| IBIS file generated by GenIBIS.pl Version 3.07
|   am35xxzcn
[IBIS ver]   4.1
[File name]   sprm451.ibs
[File Rev]   1.0
[Date]   Mon May 10, 2010, 10:46:0
[Source]   Data created at Texas Instruments
[Notes]   1) IBIS spec conformance checker (IBISCK4) ran with 0 errors
   and 179 warnings.  Warnings can be waived.
[Disclaimer] Please be aware that in the absence of a written agreement,
   Texas Instruments (TI) assumes no liability for: 1) the
   accuracy of the IBIS models provided to your company, 2) the
   proper functioning of these IBIS models in your design or for
   any resulting applications, or, 3) infringement of patents,
   copyrights, or intellectual property rights resulting from
   your use of these IBIS models. TI provides IBIS models as a
   service to our customers and therefore reserves the right to
   limit distribution of the IBIS models.
[Copyright]   Property of Texas Instruments Incorporated. Unauthorised
   reproduction and/or distribution is strictly prohibited. This
   product is protected under copyright law and trade secret law
   as an unpublished work. Created 2010,(C) Copyright 2010,
   Texas Instruments Incorporated., All Rights Reserved. These
   commodities are under the U.S. Government distribution license
   control.As such,they are not to be re-exported without the
   prior approval of the U.S. Department of Commerce.
|   Component am35xxzcn
[Component]   am35xxzcn
[Manufacturer]   Texas Instruments.
[Package Model] am35xxzcn
[Package]
|   typ   min   max
R_pkg   0.6975   3.15E-1   1.08E0
L_pkg   3.5033E-009   2.66E-11   6.98E-9
C_pkg   6.86115E-013   2.23E-15   1.37E-12
[Pin]   signal_name   model_name
A2   SDRC_DQS3P   Selector_16
A3   SDRC_D25   Selector_16
A4   SDRC_STRBEN_DLY1   Selector_16
A5   SDRC_STRBEN1   Selector_3
A6   SDRC_DQS2P   Selector_16
A7   SDRC_D16   Selector_16
A8   SDRC_A12   Selector_27
A9   SDRC_A10   Selector_27
A10   SDRC_A5   Selector_27
A11   SDRC_A0   Selector_27
A12   SDRC_BA0   Selector_27
A13   SDRC_CLK   Selector_27
A14   SDRC_NCS1   Selector_27
A15   SDRC_D15   Selector_16
A16   SDRC_D14   Selector_16
A17   SDRC_DQS1N   Selector_16
A18   SDRC_STRBEN_DLY0   Selector_16
A19   SDRC_STRBEN0   Selector_3
A20   SDRC_DQS0N   Selector_16
A21   SDRC_D1   Selector_16
A22   MCBSP4_FSX   Selector_25
A23   MCBSP4_DR   Selector_25
A24   MCBSP3_CLKX   Selector_25
AA1   SYS_BOOT1   Selector_26
AA2   SYS_BOOT2   Selector_26
AA3   SYS_BOOT3   Selector_26
AA7   RMII_RXD1   Selector_12
AA9   MMC1_CLK   Selector_25
AA10   MMC1_DAT3   Selector_25
AA16   MCSPI2_CS0   Selector_4
AA18   ETK_D3   Selector_8
AA19   UART1_TX   Selector_25
AA23   DSS_DATA7   Selector_8
AA24   DSS_DATA8   Selector_8
AA25   DSS_DATA9   Selector_8
AB1   SYS_BOOT4   Selector_26
AB2   SYS_BOOT5   Selector_26
AB6   CCDC_DATA6   Selector_25
AB7   RMII_CRS_DV   Selector_12
AB9   MMC1_CMD   Selector_25
AB10   MMC1_DAT4   Selector_25
AB12   MMC2_DAT0   Selector_12
AB13   MMC2_DAT4   Selector_25
AB15   MCSPI1_CS0   Selector_12
AB16   MCSPI2_SOMI   Selector_8
AB18   ETK_D2   Selector_4
AB19   ETK_D7   Selector_8
AB20   ETK_D11   Selector_8
AB24   DSS_DATA5   Selector_25
AB25   DSS_DATA6   Selector_8
AC1   SYS_BOOT6   Selector_26
AC2   SYS_BOOT7   Selector_23
AC3   SYS_BOOT8   Selector_23
AC5   CCDC_DATA2   Selector_25
AC6   CCDC_DATA7   Selector_25
AC7   RMII_RXER   Selector_12
AC9   MMC1_DAT0   Selector_25
AC10   MMC1_DAT5   Selector_25
AC12   MMC2_DAT1   Selector_12
AC13   MMC2_DAT5   Selector_25
AC15   MCSPI1_SOMI   Selector_25
AC16   MCSPI2_SIMO   Selector_8
AC18   ETK_D1   Selector_4
AC20   ETK_D10   Selector_8
AC21   ETK_D14   Selector_25
AC23   DSS_DATA2   Selector_25
AC24   DSS_DATA3   Selector_25
AC25   DSS_DATA4   Selector_25
AD1   CCDC_FIELD   Selector_25
AD2   CCDC_PCLK   Selector_25
AD3   CCDC_VD   Selector_25
AD4   CCDC_DATA0   Selector_25
AD5   CCDC_DATA3   Selector_25
AD6   RMII_MDIO_CLK   Selector_12
AD7   RMII_TXD0   Selector_12
AD8   RMII_TXEN   Selector_12
AD9   MMC1_DAT1   Selector_25
AD10   MMC1_DAT6   Selector_25
AD11   MMC2_CLK   Selector_25
AD12   MMC2_DAT2   Selector_12
AD13   MMC2_DAT6   Selector_25
AD14   MCSPI1_CS1   Selector_12
AD15   MCSPI1_SIMO   Selector_25
AD16   MCSPI2_CLK   Selector_8
AD17   ETK_CLK   Selector_4
AD18   ETK_D0   Selector_4
AD19   ETK_D6   Selector_8
AD20   ETK_D9   Selector_8
AD21   ETK_D13   Selector_25
AD22   DSS_HSYNC   Selector_12
AD23   DSS_VSYNC   Selector_12
AD24   DSS_DATA0   Selector_25
AD25   DSS_DATA1   Selector_25
AE2   CCDC_HD   Selector_25
AE3   CCDC_WEN   Selector_25
AE4   CCDC_DATA1   Selector_25
AE5   CCDC_DATA4   Selector_25
AE6   RMII_MDIO_DATA   Selector_12
AE7   RMII_TXD1   Selector_12
AE8   RMII_50MHZ_CLK   Selector_12
AE9   MMC1_DAT2   Selector_25
AE10   MMC1_DAT7   Selector_25
AE11   MMC2_CMD   Selector_12
AE12   MMC2_DAT3   Selector_12
AE13   MMC2_DAT7   Selector_25
AE14   MCSPI1_CLK   Selector_25
AE15   MCSPI1_CS2   Selector_4
AE16   MCSPI1_CS3   Selector_4
AE17   MCSPI2_CS1   Selector_8
AE18   ETK_CTL   Selector_4
AE19   ETK_D5   Selector_8
AE20   ETK_D8   Selector_8
AE21   ETK_D12   Selector_25
AE22   ETK_D15   Selector_25
AE23   DSS_PCLK   Selector_12
AE24   DSS_ACBIAS   Selector_25
B1   SDRC_D30   Selector_16
B2   SDRC_DQS3N   Selector_16
B3   SDRC_D26   Selector_16
B4   SDRC_D24   Selector_16
B5   SDRC_D22   Selector_16
B6   SDRC_DQS2N   Selector_16
B7   SDRC_D17   Selector_16
B8   SDRC_A13   Selector_27
B9   SDRC_A11   Selector_27
B10   SDRC_A6   Selector_27
B11   SDRC_A1   Selector_27
B13   SDRC_NCLK   Selector_27
B14   SDRC_NWE   Selector_27
B15   SDRC_DM1   Selector_27
B16   SDRC_D13   Selector_16
B17   SDRC_DQS1P   Selector_16
B18   SDRC_D8   Selector_16
B19   SDRC_D7   Selector_16
B20   SDRC_DQS0P   Selector_16
B21   SDRC_D0   Selector_16
B22   MCBSP4_DX   Selector_25
B23   MCBSP4_CLKX   Selector_25
B24   MCBSP3_DX   Selector_25
B25   MCBSP2_DR   Selector_25
C1   SDRC_D31   Selector_16
C2   SDRC_D28   Selector_16
C3   SDRC_D27   Selector_16
C5   SDRC_D23   Selector_16
C6   SDRC_D20   Selector_16
C8   SDRC_ODT0   Selector_3
C10   SDRC_A7   Selector_27
C11   SDRC_A2   Selector_27
C13   SDRC_BA1   Selector_27
C14   SDRC_NRAS   Selector_27
C16   SDRC_D12   Selector_16
C17   SDRC_D10   Selector_16
C19   SDRC_D6   Selector_16
C20   SDRC_D3   Selector_16
C21   SDRC_DM0   Selector_27
C23   MCBSP3_FSX   Selector_25
C24   MCBSP3_DR   Selector_25
C25   MCBSP2_CLKX   Selector_25
D1   SDRC_DM3   Selector_27
D2   SDRC_D29   Selector_16
D6   SDRC_D21   Selector_16
D7   SDRC_D18   Selector_16
D8   SDRC_A14   Selector_27
D10   SDRC_A8   Selector_27
D11   SDRC_A3   Selector_27
D13   SDRC_BA2   Selector_27
D14   SDRC_CKE0   Selector_27
D16   SDRC_D11   Selector_16
D17   SDRC_D9   Selector_16
D19   SDRC_D5   Selector_16
D20   SDRC_D2   Selector_16
D24   MCBSP2_DX   Selector_25
D25   MCBSP2_FSX   Selector_25
E1   GPMC_A3   Selector_1
E2   GPMC_A2   Selector_1
E3   GPMC_A1   Selector_1
E7   SDRC_D19   Selector_16
E8   SDRC_DM2   Selector_27
E10   SDRC_A9   Selector_27
E11   SDRC_A4   Selector_27
E13   SDRC_NCS0   Selector_27
E14   SDRC_NCAS   Selector_27
E19   SDRC_D4   Selector_16
E23   UART2_RX   Selector_12
E24   UART2_TX   Selector_12
E25   USB0_DRVVBUS   Selector_9
F1   GPMC_A9   Selector_28
F2   GPMC_A8   Selector_28
F3   GPMC_A7   Selector_28
F4   GPMC_A6   Selector_28
F6   GPMC_A5   Selector_1
F7   GPMC_A4   Selector_1
F19   UART2_RTS   Selector_12
F20   UART2_CTS   Selector_12
G1   GPMC_D4   Selector_28
G2   GPMC_D3   Selector_28
G3   GPMC_D2   Selector_28
G4   GPMC_D1   Selector_28
G5   GPMC_D0   Selector_28
G6   GPMC_A10   Selector_28
H1   GPMC_D6   Selector_28
H2   GPMC_D5   Selector_28
J1   GPMC_D11   Selector_28
J2   GPMC_D10   Selector_28
J3   GPMC_D9   Selector_28
J4   GPMC_D8   Selector_28
J5   GPMC_D7   Selector_28
K1   GPMC_D15   Selector_28
K2   GPMC_D14   Selector_28
K3   GPMC_D13   Selector_28
K4   GPMC_D12   Selector_28
K24   SYS_32K   Selector_17
K25   SYS_XTALIN   Selector_11
L1   GPMC_NCS1   Selector_28
L2   GPMC_NCS0   Selector_28
L25   HDQ_SIO   Selector_14
M1   GPMC_NCS5   Selector_28
M2   GPMC_NCS4   Selector_28
M3   GPMC_NCS3   Selector_28
M4   GPMC_NCS2   Selector_28
M24   SYS_CLKREQ   Selector_5
M25   SYS_CLKOUT2   Selector_5
N1   GPMC_CLK   Selector_6
N2   UART3_CTS_RCTX   Selector_14
N3   UART3_RTS_SD   Selector_18
N4   GPMC_NCS7   Selector_28
N5   GPMC_NCS6   Selector_28
N24   MCBSP1_CLKX   Selector_8
N25   SYS_CLKOUT1   Selector_14
P1   UART3_RX_IRRX   Selector_18
P2   UART3_TX_IRTX   Selector_18
P21   MCBSP1_FSR   Selector_8
P22   MCBSP1_DX   Selector_8
P23   MCBSP1_DR   Selector_8
P24   MCBSP1_FSX   Selector_8
P25   MCBSP_CLKS   Selector_8
R1   GPMC_NADV_ALE   Selector_20
R2   GPMC_NOE   Selector_21
R3   GPMC_NWE   Selector_21
R4   GPMC_NBE0_CLE   Selector_1
R24   JTAG_EMU1   Selector_14
R25   MCBSP1_CLKR   Selector_8
T1   GPMC_NBE1   Selector_1
T2   GPMC_NWP   Selector_1
T3   GPMC_WAIT0   Selector_22
T4   GPMC_WAIT1   Selector_19
T5   GPMC_WAIT2   Selector_19
T21   JTAG_RTCK   Selector_2
T22   JTAG_TMS_TMSC   Selector_14
T23   JTAG_TDI   Selector_15
T24   JTAG_TDO   Selector_2
T25   JTAG_EMU0   Selector_14
U1   GPMC_WAIT3   Selector_19
U21   DSS_DATA21   Selector_8
U22   DSS_DATA22   Selector_8
U23   DSS_DATA23   Selector_8
U24   JTAG_NTRST   Selector_13
U25   JTAG_TCK   Selector_13
V2   HECC1_TXD   Selector_18
V3   HECC1_RXD   Selector_18
V4   I2C1_SCL   Selector_7
V5   I2C1_SDA   Selector_7
V24   DSS_DATA19   Selector_8
V25   DSS_DATA20   Selector_8
W1   I2C2_SCL   Selector_10
W2   I2C2_SDA   Selector_10
W4   I2C3_SCL   Selector_10
W5   I2C3_SDA   Selector_10
W20   UART1_RX   Selector_25
W21   DSS_DATA14   Selector_8
W22   DSS_DATA15   Selector_8
W23   DSS_DATA16   Selector_8
W24   DSS_DATA17   Selector_8
W25   DSS_DATA18   Selector_8
Y1   SYS_NIRQ   Selector_18
Y2   SYS_NRESPWRON   Selector_24
Y3   SYS_NRESWARM   Selector_9
Y4   SYS_BOOT0   Selector_26
Y6   CCDC_DATA5   Selector_25
Y7   RMII_RXD0   Selector_12
Y18   ETK_D4   Selector_8
Y19   UART1_RTS   Selector_25
Y20   UART1_CTS   Selector_25
Y22   DSS_DATA10   Selector_8
Y23   DSS_DATA11   Selector_8
Y24   DSS_DATA12   Selector_8
Y25   DSS_DATA13   Selector_8
| Device pads which are not required to be modeled. Included for completeness
|A1   VSS   VSS.PAD
|A25   VSS   VSS.PAD
|AA12   CAP_VDD_SRAM_MPU   PASSIVE.PAD
|AA13   VDDS_SRAM_MPU   VDD.PAD
|AA15   VDDS_DPLL_MPU_USBHOST VDD.PAD
|AE1   VSS   VSS.PAD
|AE25   VSS   VSS.PAD
|B12   DDR_PADREF   OVTPOSSTL18TCG_7LM.PAD
|E16   CAP_VDD_SRAM_CORE   PASSIVE.PAD
|E17   VDDS_SRAM_CORE_BG   VDD.PAD
|F8   VDDS   VDD.PAD
|F10   VDDS   VDD.PAD
|F11   VDDS   VDD.PAD
|F13   VDDS   VDD.PAD
|F14   VREFSSTL   PASSIVE.PAD
|F16   VDDS   VDD.PAD
|F22   CAP_VDDA1P2LDO_USBPHY PASSIVE.PAD
|F23   VDDA3P3V_USBPHY   VDD.PAD
|F24   USB0_DM   COMPLEXIO.PAD
|F25   USB0_DP   COMPLEXIO.PAD
|G8   VDDS   VDD.PAD
|G10   VDDS   VDD.PAD
|G11   VDDS   VDD.PAD
|G13   VDDS   VDD.PAD
|G14   VDDS   VDD.PAD
|G16   VDDS   VDD.PAD
|G17   VDDS   VDD.PAD
|G20   VSS   VSS.PAD
|G21   VSS   VSS.PAD
|G22   VDDA1P8V_USBPHY   VDD.PAD
|G24   USB0_VBUS   COMPLEXIO.PAD
|G25   USB0_ID   COMPLEXIO.PAD
|H8   VDDS   VDD.PAD
|H9   VSS   VSS.PAD
|H10   VDD_CORE   VDD.PAD
|H11   VDD_CORE   VDD.PAD
|H12   VSS   VSS.PAD
|H13   VSS   VSS.PAD
|H14   VSS   VSS.PAD
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[Model Selector] Selector_1
Model_56 I/O,1.8V,PD
Model_57 I/O,1.8V,PU
Model_58 I/O,1.8V,PI
Model_59 I/O,3.3V,PD
Model_60 I/O,3.3V,PU
Model_61 I/O,3.3V,PI
|   Usage O#1.8V/3.3V###BC1833DV50BTPBFZP18LL_7LM.PAD
|   Base model BC1833DV50BTPBFZP18LL_7LM
[Model Selector] Selector_2
Model_10 I/O,3.3V,PD
Model_11 I/O,3.3V,PU
Model_12 I/O,3.3V,PI
Model_7 I/O,1.8V,PD
Model_8 I/O,1.8V,PU
Model_9 I/O,1.8V,PI
|   Usage IO#1.8V#NONE_LVCMOS#FAST#BSSTL18TCSCGPBFZ_7LM.PAD
|   Base model BSSTL18TCSCGPBFZ_7LM
[Model Selector] Selector_3
Model_102 3-STATE,1.8V,PI,FAST,+-10%V
Model_105 INPUT,1.8V,NONE_LVCMOS,+-10%V
Model_115 3-STATE,1.8V,PI,FAST,+-0.1V
Model_118 INPUT,1.8V,NONE_LVCMOS,+-0.1V
|   Usage IO#1.8V/3.3V#PD/PI/PU##BC1833DV40CTPBFHP18LL_7LM.PAD
|   Base model BC1833DV40CTPBFHP18LL_7LM
[Model Selector] Selector_4
Model_1 I/O,1.8V,PD
Model_2 I/O,1.8V,PU
Model_3 I/O,1.8V,PI
Model_4 I/O,3.3V,PD
Model_5 I/O,3.3V,PU
Model_6 I/O,3.3V,PI
|   Usage IO#1.8V/3.3V#PD/PI/PU##BC1833DV50BTPBFZP18LL_7LM.PAD
|   Base model BC1833DV50BTPBFZP18LL_7LM
[Model Selector] Selector_5
Model_10 I/O,3.3V,PD
Model_11 I/O,3.3V,PU
Model_12 I/O,3.3V,PI
Model_7 I/O,1.8V,PD
Model_8 I/O,1.8V,PU
Model_9 I/O,1.8V,PI
|   Usage IO#1.8V/3.3V#PD/PI/PU##BQ1833DV40DTPBFZP18LL_7LM.PAD
|   Base model BQ1833DV40DTPBFZP18LL_7LM
[Model Selector] Selector_6
Model_31 I/O,1.8V,PD
Model_32 I/O,1.8V,PU
Model_33 I/O,1.8V,PI
Model_34 I/O,3.3V,PD
Model_35 I/O,3.3V,PU
Model_36 I/O,3.3V,PI
|   Usage OD#1.8V/3.3V#PD/PI/PU##BC1833DV65ATPBFHP18LL_7LM_X50.PAD
|   Base model BC1833DV65ATPBFHP18LL_7LM_X50
[Model Selector] Selector_7
Model_19 I/O,1.8V,PD
Model_20 I/O,1.8V,PU
Model_21 I/O,1.8V,PI
Model_22 I/O,3.3V,PD
Model_23 I/O,3.3V,PU
Model_24 I/O,3.3V,PI
|   Usage IO#1.8V/3.3V#PD/PI/PU##BC1833DV40CTPBFZP18LL_7LM.PAD
|   Base model BC1833DV40CTPBFZP18LL_7LM
[Model Selector] Selector_8
Model_76 I/O,1.8V,PD
Model_77 I/O,1.8V,PU
Model_78 I/O,1.8V,PI
Model_79 I/O,3.3V,PD
Model_80 I/O,3.3V,PU
Model_81 I/O,3.3V,PI
|   Usage IO#1.8V/3.3V#PD/PI/PU##BC1833DV50BTPBFZP18LL_7LM_X50.PAD
|   Base model BC1833DV50BTPBFZP18LL_7LM_X50
[Model Selector] Selector_9
Model_94 I/O,1.8V,PD
Model_95 I/O,1.8V,PU
Model_96 I/O,1.8V,PI
Model_97 I/O,3.3V,PD
Model_98 I/O,3.3V,PU
Model_99 I/O,3.3V,PI
|   Usage IO#1.8V/3.3V#PD/PI/PU##BC1833DV65ATPBFHP18LL_7LM_X50.PAD
|   Base model BC1833DV65ATPBFHP18LL_7LM_X50
[Model Selector] Selector_10
Model_19 I/O,1.8V,PD
Model_20 I/O,1.8V,PU
Model_21 I/O,1.8V,PI
Model_22 I/O,3.3V,PD
Model_23 I/O,3.3V,PU
Model_24 I/O,3.3V,PI
|   Usage I#1.8V###IOSCHF18CVSHY_7LM.PAD
|   Base model IOSCHF18CVSHY_7LM
[Model Selector] Selector_11
Model_37 INPUT,1.8V
|   Usage IO#1.8V/3.3V#PD/PI/PU##BC1833DV40CTPBFHP18LL_7LM_X50.PAD
|   Base model BC1833DV40CTPBFHP18LL_7LM_X50
[Model Selector] Selector_12
Model_70 I/O,1.8V,PD
Model_71 I/O,1.8V,PU
Model_72 I/O,1.8V,PI
Model_73 I/O,3.3V,PD
Model_74 I/O,3.3V,PU
Model_75 I/O,3.3V,PI
|   Usage I#1.8V/3.3V#PD/PI/PU##IC1833DVTPBFZP18LL_7LM.PAD
|   Base model IC1833DVTPBFZP18LL_7LM
[Model Selector] Selector_13
Model_13 INPUT,1.8V,PD
Model_14 INPUT,1.8V,PU
Model_15 INPUT,1.8V,PI
Model_16 INPUT,3.3V,PD
Model_17 INPUT,3.3V,PU
Model_18 INPUT,3.3V,PI
|   Usage IO#1.8V/3.3V#PD/PI/PU##BC1833DV50BTPBFHP18LL_7LM.PAD
|   Base model BC1833DV50BTPBFHP18LL_7LM
[Model Selector] Selector_14
Model_134 I/O,1.8V,PD
Model_135 I/O,1.8V,PU
Model_136 I/O,1.8V,PI
Model_137 I/O,3.3V,PD
Model_138 I/O,3.3V,PU
Model_139 I/O,3.3V,PI
|   Usage I#1.8V/3.3V#PD/PI/PU##IC1833DVTPBFHP18LL_7LM.PAD
|   Base model IC1833DVTPBFHP18LL_7LM
[Model Selector] Selector_15
Model_44 INPUT,1.8V,PD
Model_45 INPUT,1.8V,PU
Model_46 INPUT,1.8V,PI
Model_47 INPUT,3.3V,PD
Model_48 INPUT,3.3V,PU
Model_49 INPUT,3.3V,PI
|   Usage IO#1.8V#FULL_SSTL/HALF_SSTL/NONE_SSTL#FAST#BSSTL18TCSCGPBFZ_7LM.PAD
|   Base model BSSTL18TCSCGPBFZ_7LM
[Model Selector] Selector_16
Model_100 INPUT,1.8V,HALF_SSTL,+-10%V
Model_102 3-STATE,1.8V,PI,FAST,+-10%V
Model_104 INPUT,1.8V,FULL_SSTL,+-10%V
Model_107 INPUT,1.8V,NONE_SSTL,+-10%V
Model_113 INPUT,1.8V,HALF_SSTL,+-0.1V
Model_115 3-STATE,1.8V,PI,FAST,+-0.1V
Model_117 INPUT,1.8V,FULL_SSTL,+-0.1V
Model_120 INPUT,1.8V,NONE_SSTL,+-0.1V
|   Usage I#1.8V/3.3V#PD/PI/PU##IQ1833DVTPBFZP18LL_7LM.PAD
|   Base model IQ1833DVTPBFZP18LL_7LM
[Model Selector] Selector_17
Model_82 INPUT,1.8V,PD
Model_83 INPUT,1.8V,PU
Model_84 INPUT,1.8V,PI
Model_85 INPUT,3.3V,PD
Model_86 INPUT,3.3V,PU
Model_87 INPUT,3.3V,PI
|   Usage IO#1.8V/3.3V#PD/PI/PU##BC1833DV50BTPBFHP18LL_7LM_X50.PAD
|   Base model BC1833DV50BTPBFHP18LL_7LM_X50
[Model Selector] Selector_18
Model_62 I/O,1.8V,PD
Model_63 I/O,1.8V,PU
Model_64 I/O,1.8V,PI
Model_65 I/O,3.3V,PD
Model_66 I/O,3.3V,PU
Model_67 I/O,3.3V,PI
|   Usage IO#1.8V/3.3V#PD/PI/PU##BQ1833DV40DTPBFHP18LL_7LM_X50.PAD
|   Base model BQ1833DV40DTPBFHP18LL_7LM_X50
[Model Selector] Selector_19
Model_50 I/O,1.8V,PD
Model_51 I/O,1.8V,PU
Model_52 I/O,1.8V,PI
Model_53 I/O,3.3V,PD
Model_54 I/O,3.3V,PU
Model_55 I/O,3.3V,PI
|   Usage O#1.8V/3.3V###BQ1833DV40DTPBFZP18LL_7LM_X50.PAD
|   Base model BQ1833DV40DTPBFZP18LL_7LM_X50
[Model Selector] Selector_20
Model_56 I/O,1.8V,PD
Model_57 I/O,1.8V,PU
Model_58 I/O,1.8V,PI
Model_59 I/O,3.3V,PD
Model_60 I/O,3.3V,PU
Model_61 I/O,3.3V,PI
|   Usage O#1.8V/3.3V###BQ1833DV40DTPBFHP18LL_7LM_X50.PAD
|   Base model BQ1833DV40DTPBFHP18LL_7LM_X50
[Model Selector] Selector_21
Model_50 I/O,1.8V,PD
Model_51 I/O,1.8V,PU
Model_52 I/O,1.8V,PI
Model_53 I/O,3.3V,PD
Model_54 I/O,3.3V,PU
Model_55 I/O,3.3V,PI
|   Usage I#1.8V/3.3V#PD/PI/PU##BQ1833DV40DTPBFHP18LL_7LM_X50.PAD
|   Base model BQ1833DV40DTPBFHP18LL_7LM_X50
[Model Selector] Selector_22
Model_50 I/O,1.8V,PD
Model_51 I/O,1.8V,PU
Model_52 I/O,1.8V,PI
Model_53 I/O,3.3V,PD
Model_54 I/O,3.3V,PU
Model_55 I/O,3.3V,PI
|   Usage I#1.8V/3.3V#PD/PI/PU##BQ1833DV50BTPBFZP18LL_7LM_X50.PAD
|   Base model BQ1833DV50BTPBFZP18LL_7LM_X50
[Model Selector] Selector_23
Model_88 I/O,1.8V,PD
Model_89 I/O,1.8V,PU
Model_90 I/O,1.8V,PI
Model_91 I/O,3.3V,PD
Model_92 I/O,3.3V,PU
Model_93 I/O,3.3V,PI
|   Usage I#1.8V/3.3V###IHHV1833DVTP18_7LM.PAD
|   Base model IHHV1833DVTP18_7LM
[Model Selector] Selector_24
Model_68 INPUT,1.8V
Model_69 INPUT,3.3V
|   Usage IO#1.8V/3.3V#PD/PI/PU##BC1833DV40CTPBFZP18LL_7LM_X50.PAD
|   Base model BC1833DV40CTPBFZP18LL_7LM_X50
[Model Selector] Selector_25
Model_38 I/O,1.8V,PD
Model_39 I/O,1.8V,PU
Model_40 I/O,1.8V,PI
Model_41 I/O,3.3V,PD
Model_42 I/O,3.3V,PU
Model_43 I/O,3.3V,PI
|   Usage IO#1.8V/3.3V#PD/PI/PU##BQ1833DV50BTPBFZP18LL_7LM_X50.PAD
|   Base model BQ1833DV50BTPBFZP18LL_7LM_X50
[Model Selector] Selector_26
Model_88 I/O,1.8V,PD
Model_89 I/O,1.8V,PU
Model_90 I/O,1.8V,PI
Model_91 I/O,3.3V,PD
Model_92 I/O,3.3V,PU
Model_93 I/O,3.3V,PI
|   Usage O#1.8V##FAST#BSSTL18TCSCGPBFZ_7LM.PAD
|   Base model BSSTL18TCSCGPBFZ_7LM
[Model Selector] Selector_27
Model_102 3-STATE,1.8V,PI,FAST,+-10%V
Model_115 3-STATE,1.8V,PI,FAST,+-0.1V
|   Usage IO#1.8V/3.3V#PD/PI/PU##BQ1833DV40DTPBFHP18LL_7LM.PAD
|   Base model BQ1833DV40DTPBFHP18LL_7LM
[Model Selector] Selector_28
Model_25 I/O,1.8V,PD
Model_26 I/O,1.8V,PU
Model_27 I/O,1.8V,PI
Model_28 I/O,3.3V,PD
Model_29 I/O,3.3V,PU
Model_30 I/O,3.3V,PI
| Package model definition
[Define Package Model]  am35xxzcn
[Manufacturer]   Texas Instruments.
[OEM]   Texas Instruments.
[Description]   am35xxzcn package model generated by GenIBIS.pl
[Number Of Pins]   287
[Pin Numbers]
A2   | 1 SDRC_DQS3P   IO
A3   | 2 SDRC_D25   IO
A4   | 3 SDRC_STRBEN_DLY1   IO
A5   | 4 SDRC_STRBEN1   IO
A6   | 5 SDRC_DQS2P   IO
A7   | 6 SDRC_D16   IO
A8   | 7 SDRC_A12   O
A9   | 8 SDRC_A10   O
A10   | 9 SDRC_A5   O
A11   | 10 SDRC_A0   O
A12   | 11 SDRC_BA0   O
A13   | 12 SDRC_CLK   O
A14   | 13 SDRC_NCS1   O
A15   | 14 SDRC_D15   IO
A16   | 15 SDRC_D14   IO
A17   | 16 SDRC_DQS1N   IO
A18   | 17 SDRC_STRBEN_DLY0   IO
A19   | 18 SDRC_STRBEN0   IO
A20   | 19 SDRC_DQS0N   IO
A21   | 20 SDRC_D1   IO
A22   | 21 MCBSP4_FSX   IO
A23   | 22 MCBSP4_DR   IO
A24   | 23 MCBSP3_CLKX   IO
AA1   | 24 SYS_BOOT1   IO
AA2   | 25 SYS_BOOT2   IO
AA3   | 26 SYS_BOOT3   IO
AA7   | 27 RMII_RXD1   IO
AA9   | 28 MMC1_CLK   IO
AA10   | 29 MMC1_DAT3   IO
AA16   | 30 MCSPI2_CS0   IO
AA18   | 31 ETK_D3   IO
AA19   | 32 UART1_TX   IO
AA23   | 33 DSS_DATA7   IO
AA24   | 34 DSS_DATA8   IO
AA25   | 35 DSS_DATA9   IO
AB1   | 36 SYS_BOOT4   IO
AB2   | 37 SYS_BOOT5   IO
AB6   | 38 CCDC_DATA6   IO
AB7   | 39 RMII_CRS_DV   IO
AB9   | 40 MMC1_CMD   IO
AB10   | 41 MMC1_DAT4   IO
AB12   | 42 MMC2_DAT0   IO
AB13   | 43 MMC2_DAT4   IO
AB15   | 44 MCSPI1_CS0   IO
AB16   | 45 MCSPI2_SOMI   IO
AB18   | 46 ETK_D2   IO
AB19   | 47 ETK_D7   IO
AB20   | 48 ETK_D11   IO
AB24   | 49 DSS_DATA5   IO
AB25   | 50 DSS_DATA6   IO
AC1   | 51 SYS_BOOT6   IO
AC2   | 52 SYS_BOOT7   I
AC3   | 53 SYS_BOOT8   I
AC5   | 54 CCDC_DATA2   IO
AC6   | 55 CCDC_DATA7   IO
AC7   | 56 RMII_RXER   IO
AC9   | 57 MMC1_DAT0   IO
AC10   | 58 MMC1_DAT5   IO
AC12   | 59 MMC2_DAT1   IO
AC13   | 60 MMC2_DAT5   IO
AC15   | 61 MCSPI1_SOMI   IO
AC16   | 62 MCSPI2_SIMO   IO
AC18   | 63 ETK_D1   IO
AC20   | 64 ETK_D10   IO
AC21   | 65 ETK_D14   IO
AC23   | 66 DSS_DATA2   IO
AC24   | 67 DSS_DATA3   IO
AC25   | 68 DSS_DATA4   IO
AD1   | 69 CCDC_FIELD   IO
AD2   | 70 CCDC_PCLK   IO
AD3   | 71 CCDC_VD   IO
AD4   | 72 CCDC_DATA0   IO
AD5   | 73 CCDC_DATA3   IO
AD6   | 74 RMII_MDIO_CLK   IO
AD7   | 75 RMII_TXD0   IO
AD8   | 76 RMII_TXEN   IO
AD9   | 77 MMC1_DAT1   IO
AD10   | 78 MMC1_DAT6   IO
AD11   | 79 MMC2_CLK   IO
AD12   | 80 MMC2_DAT2   IO
AD13   | 81 MMC2_DAT6   IO
AD14   | 82 MCSPI1_CS1   IO
AD15   | 83 MCSPI1_SIMO   IO
AD16   | 84 MCSPI2_CLK   IO
AD17   | 85 ETK_CLK   IO
AD18   | 86 ETK_D0   IO
AD19   | 87 ETK_D6   IO
AD20   | 88 ETK_D9   IO
AD21   | 89 ETK_D13   IO
AD22   | 90 DSS_HSYNC   IO
AD23   | 91 DSS_VSYNC   IO
AD24   | 92 DSS_DATA0   IO
AD25   | 93 DSS_DATA1   IO
AE2   | 94 CCDC_HD   IO
AE3   | 95 CCDC_WEN   IO
AE4   | 96 CCDC_DATA1   IO
AE5   | 97 CCDC_DATA4   IO
AE6   | 98 RMII_MDIO_DATA   IO
AE7   | 99 RMII_TXD1   IO
AE8   | 100 RMII_50MHZ_CLK   IO
AE9   | 101 MMC1_DAT2   IO
AE10   | 102 MMC1_DAT7   IO
AE11   | 103 MMC2_CMD   IO
AE12   | 104 MMC2_DAT3   IO
AE13   | 105 MMC2_DAT7   IO
AE14   | 106 MCSPI1_CLK   IO
AE15   | 107 MCSPI1_CS2   IO
AE16   | 108 MCSPI1_CS3   IO
AE17   | 109 MCSPI2_CS1   IO
AE18   | 110 ETK_CTL   IO
AE19   | 111 ETK_D5   IO
AE20   | 112 ETK_D8   IO
AE21   | 113 ETK_D12   IO
AE22   | 114 ETK_D15   IO
AE23   | 115 DSS_PCLK   IO
AE24   | 116 DSS_ACBIAS   IO
B1   | 117 SDRC_D30   IO
B2   | 118 SDRC_DQS3N   IO
B3   | 119 SDRC_D26   IO
B4   | 120 SDRC_D24   IO
B5   | 121 SDRC_D22   IO
B6   | 122 SDRC_DQS2N   IO
B7   | 123 SDRC_D17   IO
B8   | 124 SDRC_A13   O
B9   | 125 SDRC_A11   O
B10   | 126 SDRC_A6   O
B11   | 127 SDRC_A1   O
B13   | 128 SDRC_NCLK   O
B14   | 129 SDRC_NWE   O
B15   | 130 SDRC_DM1   O
B16   | 131 SDRC_D13   IO
B17   | 132 SDRC_DQS1P   IO
B18   | 133 SDRC_D8   IO
B19   | 134 SDRC_D7   IO
B20   | 135 SDRC_DQS0P   IO
B21   | 136 SDRC_D0   IO
B22   | 137 MCBSP4_DX   IO
B23   | 138 MCBSP4_CLKX   IO
B24   | 139 MCBSP3_DX   IO
B25   | 140 MCBSP2_DR   IO
C1   | 141 SDRC_D31   IO
C2   | 142 SDRC_D28   IO
C3   | 143 SDRC_D27   IO
C5   | 144 SDRC_D23   IO
C6   | 145 SDRC_D20   IO
C8   | 146 SDRC_ODT0   IO
C10   | 147 SDRC_A7   O
C11   | 148 SDRC_A2   O
C13   | 149 SDRC_BA1   O
C14   | 150 SDRC_NRAS   O
C16   | 151 SDRC_D12   IO
C17   | 152 SDRC_D10   IO
C19   | 153 SDRC_D6   IO
C20   | 154 SDRC_D3   IO
C21   | 155 SDRC_DM0   O
C23   | 156 MCBSP3_FSX   IO
C24   | 157 MCBSP3_DR   IO
C25   | 158 MCBSP2_CLKX   IO
D1   | 159 SDRC_DM3   O
D2   | 160 SDRC_D29   IO
D6   | 161 SDRC_D21   IO
D7   | 162 SDRC_D18   IO
D8   | 163 SDRC_A14   O
D10   | 164 SDRC_A8   O
D11   | 165 SDRC_A3   O
D13   | 166 SDRC_BA2   O
D14   | 167 SDRC_CKE0   O
D16   | 168 SDRC_D11   IO
D17   | 169 SDRC_D9   IO
D19   | 170 SDRC_D5   IO
D20   | 171 SDRC_D2   IO
D24   | 172 MCBSP2_DX   IO
D25   | 173 MCBSP2_FSX   IO
E1   | 174 GPMC_A3   IO
E2   | 175 GPMC_A2   IO
E3   | 176 GPMC_A1   IO
E7   | 177 SDRC_D19   IO
E8   | 178 SDRC_DM2   O
E10   | 179 SDRC_A9   O
E11   | 180 SDRC_A4   O
E13   | 181 SDRC_NCS0   O
E14   | 182 SDRC_NCAS   O
E19   | 183 SDRC_D4   IO
E23   | 184 UART2_RX   IO
E24   | 185 UART2_TX   IO
E25   | 186 USB0_DRVVBUS   IO
F1   | 187 GPMC_A9   IO
F2   | 188 GPMC_A8   IO
F3   | 189 GPMC_A7   IO
F4   | 190 GPMC_A6   IO
F6   | 191 GPMC_A5   IO
F7   | 192 GPMC_A4   IO
F19   | 193 UART2_RTS   IO
F20   | 194 UART2_CTS   IO
G1   | 195 GPMC_D4   IO
G2   | 196 GPMC_D3   IO
G3   | 197 GPMC_D2   IO
G4   | 198 GPMC_D1   IO
G5   | 199 GPMC_D0   IO
G6   | 200 GPMC_A10   IO
H1   | 201 GPMC_D6   IO
H2   | 202 GPMC_D5   IO
J1   | 203 GPMC_D11   IO
J2   | 204 GPMC_D10   IO
J3   | 205 GPMC_D9   IO
J4   | 206 GPMC_D8   IO
J5   | 207 GPMC_D7   IO
K1   | 208 GPMC_D15   IO
K2   | 209 GPMC_D14   IO
K3   | 210 GPMC_D13   IO
K4   | 211 GPMC_D12   IO
K24   | 212 SYS_32K   I
K25   | 213 SYS_XTALIN   I
L1   | 214 GPMC_NCS1   IO
L2   | 215 GPMC_NCS0   IO
L25   | 216 HDQ_SIO   IO
M1   | 217 GPMC_NCS5   IO
M2   | 218 GPMC_NCS4   IO
M3   | 219 GPMC_NCS3   IO
M4   | 220 GPMC_NCS2   IO
M24   | 221 SYS_CLKREQ   IO
M25   | 222 SYS_CLKOUT2   IO
N1   | 223 GPMC_CLK   IO
N2   | 224 UART3_CTS_RCTX   IO
N3   | 225 UART3_RTS_SD   IO
N4   | 226 GPMC_NCS7   IO
N5   | 227 GPMC_NCS6   IO
N24   | 228 MCBSP1_CLKX   IO
N25   | 229 SYS_CLKOUT1   IO
P1   | 230 UART3_RX_IRRX   IO
P2   | 231 UART3_TX_IRTX   IO
P21   | 232 MCBSP1_FSR   IO
P22   | 233 MCBSP1_DX   IO
P23   | 234 MCBSP1_DR   IO
P24   | 235 MCBSP1_FSX   IO
P25   | 236 MCBSP_CLKS   IO
R1   | 237 GPMC_NADV_ALE   O
R2   | 238 GPMC_NOE   O
R3   | 239 GPMC_NWE   O
R4   | 240 GPMC_NBE0_CLE   IO
R24   | 241 JTAG_EMU1   IO
R25   | 242 MCBSP1_CLKR   IO
T1   | 243 GPMC_NBE1   IO
T2   | 244 GPMC_NWP   IO
T3   | 245 GPMC_WAIT0   I
T4   | 246 GPMC_WAIT1   IO
T5   | 247 GPMC_WAIT2   IO
T21   | 248 JTAG_RTCK   O
T22   | 249 JTAG_TMS_TMSC   IO
T23   | 250 JTAG_TDI   I
T24   | 251 JTAG_TDO   O
T25   | 252 JTAG_EMU0   IO
U1   | 253 GPMC_WAIT3   IO
U21   | 254 DSS_DATA21   IO
U22   | 255 DSS_DATA22   IO
U23   | 256 DSS_DATA23   IO
U24   | 257 JTAG_NTRST   I
U25   | 258 JTAG_TCK   I
V2   | 259 HECC1_TXD   IO
V3   | 260 HECC1_RXD   IO
V4   | 261 I2C1_SCL   OD
V5   | 262 I2C1_SDA   OD
V24   | 263 DSS_DATA19   IO
V25   | 264 DSS_DATA20   IO
W1   | 265 I2C2_SCL   IO
W2   | 266 I2C2_SDA   IO
W4   | 267 I2C3_SCL   IO
W5   | 268 I2C3_SDA   IO
W20   | 269 UART1_RX   IO
W21   | 270 DSS_DATA14   IO
W22   | 271 DSS_DATA15   IO
W23   | 272 DSS_DATA16   IO
W24   | 273 DSS_DATA17   IO
W25   | 274 DSS_DATA18   IO
Y1   | 275 SYS_NIRQ   IO
Y2   | 276 SYS_NRESPWRON   I
Y3   | 277 SYS_NRESWARM   IO
Y4   | 278 SYS_BOOT0   IO
Y6   | 279 CCDC_DATA5   IO
Y7   | 280 RMII_RXD0   IO
Y18   | 281 ETK_D4   IO
Y19   | 282 UART1_RTS   IO
Y20   | 283 UART1_CTS   IO
Y22   | 284 DSS_DATA10   IO
Y23   | 285 DSS_DATA11   IO
Y24   | 286 DSS_DATA12   IO
Y25   | 287 DSS_DATA13   IO
[Model Data]
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[End Model Data]
[End Package Model]
| Models and submodels in the file (115): Model_1 (I/O), Model_2 (I/O), Model_3 (I/O), Model_4 (I/O), Model_5 (I/O), Model_6 (I/O), Model_7 (I/O), Model_8 (I/O), Model_9 (I/O), Model_10 (I/O), Model_11 (I/O), Model_12 (I/O), Model_13 (Input), Model_14 (Input), Model_15 (Input), Model_16 (Input), Model_17 (Input), Model_18 (Input), Model_19 (I/O), Model_20 (I/O), Model_21 (I/O), Model_22 (I/O), Model_23 (I/O), Model_24 (I/O), Model_25 (I/O), Model_26 (I/O), Model_27 (I/O), Model_28 (I/O), Model_29 (I/O), Model_30 (I/O), Model_31 (I/O), Model_32 (I/O), Model_33 (I/O), Model_34 (I/O), Model_35 (I/O), Model_36 (I/O), Model_37 (Input), Model_38 (I/O), Model_39 (I/O), Model_40 (I/O), Model_41 (I/O), Model_42 (I/O), Model_43 (I/O), Model_44 (Input), Model_45 (Input), Model_46 (Input), Model_47 (Input), Model_48 (Input), Model_49 (Input), Model_50 (I/O), Model_51 (I/O), Model_52 (I/O), Model_53 (I/O), Model_54 (I/O), Model_55 (I/O), Model_56 (I/O), Model_57 (I/O), Model_58 (I/O), Model_59 (I/O), Model_60 (I/O), Model_61 (I/O), Model_62 (I/O), Model_63 (I/O), Model_64 (I/O), Model_65 (I/O), Model_66 (I/O), Model_67 (I/O), Model_68 (Input), Model_69 (Input), Model_70 (I/O), Model_71 (I/O), Model_72 (I/O), Model_73 (I/O), Model_74 (I/O), Model_75 (I/O), Model_76 (I/O), Model_77 (I/O), Model_78 (I/O), Model_79 (I/O), Model_80 (I/O)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
